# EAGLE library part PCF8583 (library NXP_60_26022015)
Clock and calendar with 240 x 8-bit RAM The PCF8583 is a clock and calendar chip, based on a 2048 bit static CMOS RAM organized as 256 words by 8 bits. Addresses and data are transferred serially via the two-line bidirectional I2C-bus. The built-in word address register is incremented automatically after each written or read data byte. Address pin A0 is used for programming the hardware address, allowing the connection of two devices to the bus without additional hardware. The built-in 32.768 kHz oscillator circuit and the first 8 bytes of the RAM are used for the clock, calendar, and counter functions. The next 8 bytes can be programmed as alarm registers or used as free RAM space. The remaining 240 bytes are free RAM locations. AAL Eindhoven MK
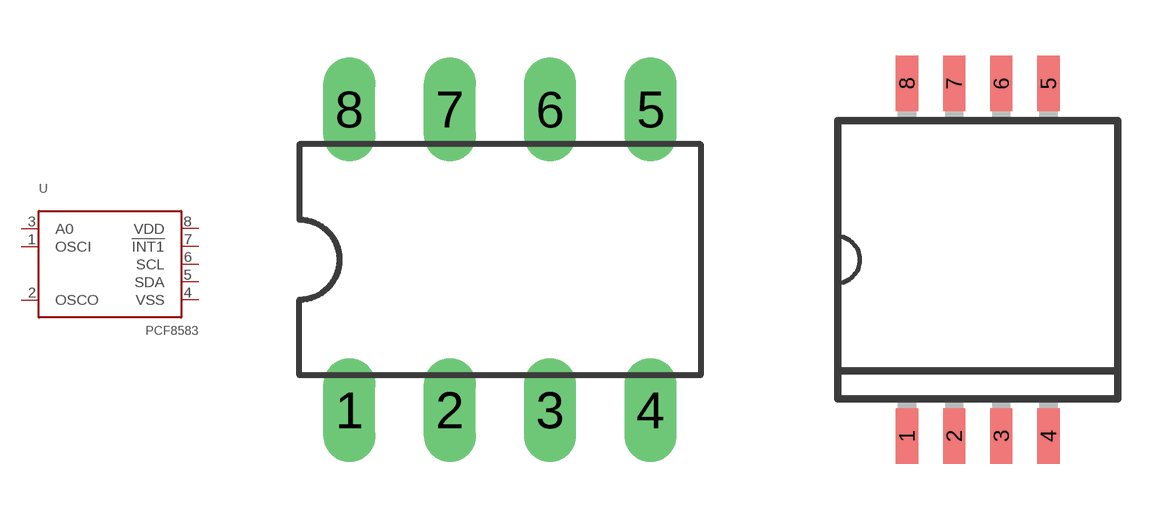
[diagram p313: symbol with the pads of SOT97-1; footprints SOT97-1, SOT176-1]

Designator prefix U

## PCF8583P  [SOT97-1]
1  OSCI  pas
2  OSCO  pas
3  A0  pwr
4  VSS  pwr
5  SDA
6  SCL  in
7  !INT1!  out
8  VDD  pwr

## PCF8583T  [SOT176-1]
Pads as for SOT97-1

## PCF8583BS  [SOT662-1]
2  OSCI  pas
3  OSCO  pas
4  A0  pwr
5  VSS  pwr
12  SDA
13  SCL  in
14  !INT1!  out
15  VDD  pwr

## Footprint SOT97-1 (pad centres in mm)
Dual In Line Package
drill 0.813 long: 1 -3.81,-3.81; 2 -1.27,-3.81; 3 1.27,-3.81; 4 3.81,-3.81; 5 3.81,3.81; 6 1.27,3.81; 7 -1.27,3.81; 8 -3.81,3.81

## Footprint SOT176-1 (pad centres in mm)
SOT176-1 SO8: plastic small outline package; 8 leads; body width 7.5 mm JEDEC: -- IEC: --
smd 0.6 x 1.5: 1 -1.905,-4.75; 2 -0.635,-4.75; 3 0.635,-4.75; 4 1.905,-4.75; 5 1.905,4.75; 6 0.635,4.75; 7 -0.635,4.75; 8 -1.905,4.75

## Footprint SOT662-1 (pad centres in mm)
SOT662-1 HVQFN20: plastic thermal enhanced very thin quad flat package; no leads; 20 terminals; body 5 x 5 x 0.85 mm JEDEC: MO-220 IEC: -- JEITA: --
smd 1.1 x 0.3: 1 -2.45,1.3; 2 -2.45,0.65; 3 -2.45,0; 4 -2.45,-0.65; 5 -2.45,-1.3; 11 2.45,-1.3; 12 2.45,-0.65; 13 2.45,0; 14 2.45,0.65; 15 2.45,1.3
smd 0.3 x 1.1: 6 -1.3,-2.45; 7 -0.65,-2.45; 8 0,-2.45; 9 0.65,-2.45; 10 1.3,-2.45; 16 1.3,2.45; 17 0.65,2.45; 18 0,2.45; 19 -0.65,2.45; 20 -1.3,2.45
smd 3 x 3: CP 0,0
